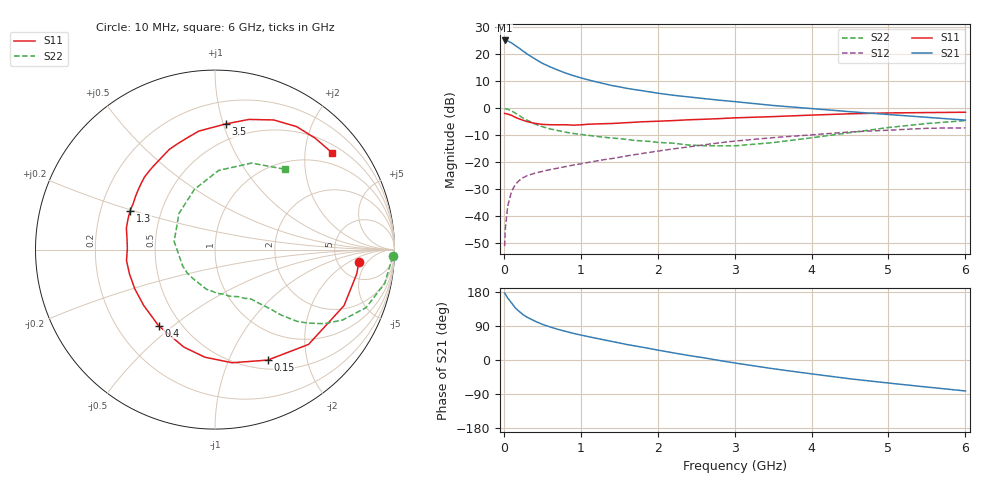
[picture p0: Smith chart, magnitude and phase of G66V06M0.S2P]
! SIEMENS Small Signal Semiconductors
! BFG193
! Si NPN RF Bipolar Junction Transistor in SOT223
! VCE = 6 V  IC = 6 mA
! Common Emitter S-Parameters:  August  1996
# GHz  S  MA  R  50
!  f  S11  S21  S12  S22
! GHz  MAG  ANG  MAG  ANG  MAG  ANG  MAG  ANG
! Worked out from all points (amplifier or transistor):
!   36 points, 10 MHz to 6 GHz, reference 50 ohm
!   highest |S21| = 25.1 dB at 10 MHz (marker M1)
!   |S21| within 3 dB of that: start of sweep to 206 MHz
!   unconditionally stable (mu >= 1): 1.078 GHz to 2.509 GHz
!   at 250 MHz: K = 0.38, MSG = 23.5 dB, |S12| = -25.7 dB
!   at 1.4 GHz: K = 1.08, MAG = 11.8 dB, |S12| = -18.6 dB
!   at 6 GHz: K = 0.86, MSG = 1.4 dB, |S12| = -7.2 dB
!   S11 on the Smith chart (normalised r, x): 10 MHz: 8.02, -3.05; 150 MHz: 0.61, -1.40; 400 MHz: 0.38, -0.44; 1.3 GHz: 0.33, +0.19; 3.5 GHz: 0.37, +1.02; 6 GHz: 0.69, +2.63
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0.01  0.8038 -4.8  18.09 176.4  0.0028 90.3  0.9897 -2.2
0.02  0.8017 -9.6  18.03 174.1  0.006 85.4  0.981 -4.6
0.05  0.7837 -23.5  17.67 163.3  0.0154 77.9  0.9639 -11.3
0.1  0.7421 -45.4  16.3 150.6  0.0289 69.2  0.9016 -21.0
0.15  0.682 -64.5  14.53 137.3  0.0389 60.1  0.8129 -28.8
0.2  0.6376 -81.4  12.99 128.1  0.0461 54.7  0.7363 -34.1
0.25  0.6021 -95.4  11.49 119.7  0.0518 50.4  0.6612 -38.3
0.3  0.57 -107.8  10.22 113.1  0.0564 47.7  0.6065 -41.2
0.4  0.5278 -126.6  8.289 102.9  0.0629 43.9  0.5157 -44.8
0.5  0.5045 -142.1  6.847 94.1  0.0679 42.6  0.4562 -46.8
0.6  0.4975 -154.0  5.879 87.3  0.0734 42.1  0.4175 -48.7
0.7  0.4954 -164.1  5.13 81.1  0.0779 42.0  0.388 -50.6
0.9  0.4884 179.1  4.053 70.5  0.0889 42.4  0.3429 -53.6
1.1  0.5082 166.3  3.358 61.6  0.0998 42.8  0.316 -59.1
1.3  0.5197 155.6  2.867 53.2  0.1121 42.6  0.2913 -64.1
1.6  0.5435 141.6  2.343 40.8  0.1315 40.9  0.2662 -74.7
2.2  0.5926 120.3  1.748 19.0  0.1773 34.5  0.2264 -101.9
2.8  0.6452 102.9  1.417 -1.2  0.2295 24.9  0.2024 -139.4
3.5  0.7028 85.1  1.13 -23.0  0.2868 9.9  0.2322 168.7
4.5  0.7931 65.6  0.867 -49.6  0.3655 -10.4  0.3548 108.8
5.5  0.8347 48.1  0.682 -71.4  0.4269 -36.0  0.5234 67.1
6  0.8468 39.5  0.605 -81.7  0.4354 -50.7  0.5927 49.1
